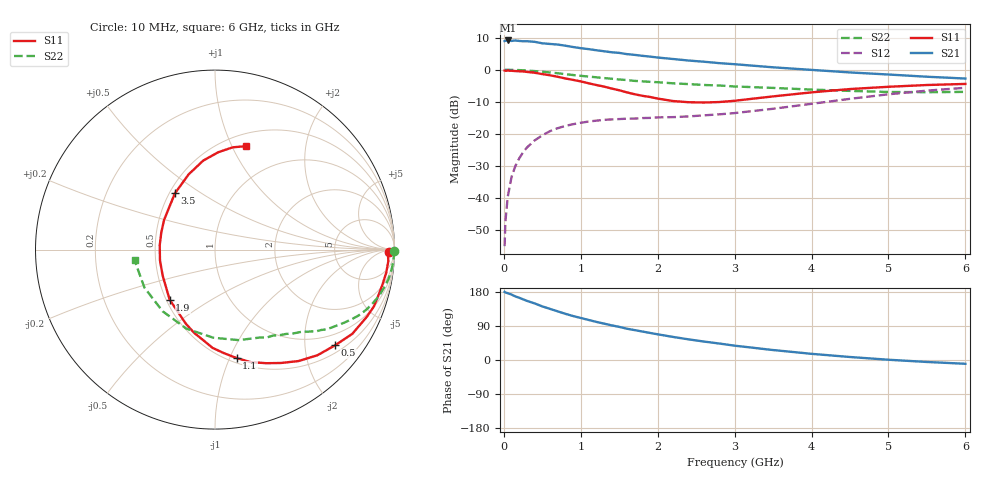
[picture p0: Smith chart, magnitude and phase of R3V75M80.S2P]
! SIEMENS Small Signal Semiconductors
! BFR181
! Si NPN RF Bipolar Junction Transistor in SOT23
! VCE = 0.75 V  IC = 0.8 mA
! Common Emitter S-Parameters:  May  1996
# GHz  S  MA  R  50
!  f  S11  S21  S12  S22
! GHz  MAG  ANG  MAG  ANG  MAG  ANG  MAG  ANG
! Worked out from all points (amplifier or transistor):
!   36 points, 10 MHz to 6 GHz, reference 50 ohm
!   highest |S21| = 9.1 dB at 50 MHz (marker M1)
!   |S21| within 3 dB of that: start of sweep to 1.189 GHz
!   unconditionally stable (mu >= 1): 2.027 GHz to 4.167 GHz
!   at 250 MHz: K = 0.15, MSG = 17.3 dB, |S12| = -25.7 dB
!   at 1.4 GHz: K = 0.74, MSG = 10.4 dB, |S12| = -15.5 dB
!   at 6 GHz: K = 0.95, MSG = 1.4 dB, |S12| = -5.6 dB
!   S11 on the Smith chart (normalised r, x): 10 MHz: 55, -25; 500 MHz: 0.68, -2.70; 1.1 GHz: 0.54, -1.06; 1.9 GHz: 0.52, -0.34; 3.5 GHz: 0.53, +0.39; 6 GHz: 0.63, +1.13
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0.01  0.9703 -0.8  2.791 179.7  0.0018 94.1  0.9983 -0.4
0.02  0.9638 -1.4  2.821 178.4  0.0043 84.0  0.9957 -0.8
0.05  0.9678 -3.8  2.852 176.2  0.0104 86.8  0.9971 -2.0
0.1  0.9627 -7.7  2.803 172.7  0.0215 84.2  0.9952 -3.9
0.15  0.9528 -12.0  2.848 167.7  0.0318 81.7  0.9907 -6.1
0.2  0.9454 -15.8  2.802 164.2  0.0418 78.9  0.9854 -7.9
0.3  0.9249 -23.9  2.776 156.1  0.0616 74.6  0.9703 -11.7
0.4  0.8977 -31.5  2.716 149.4  0.0794 69.2  0.952 -15.4
0.5  0.8554 -38.6  2.576 141.4  0.0954 64.6  0.9291 -18.7
0.7  0.7763 -53.1  2.463 128.4  0.1231 56.7  0.8809 -24.6
0.8  0.7309 -59.8  2.364 121.9  0.1337 52.9  0.8536 -27.1
1.1  0.6162 -78.7  2.092 105.8  0.1563 44.6  0.7829 -33.6
1.3  0.5473 -91.5  1.939 96.1  0.1659 40.6  0.7424 -37.1
1.6  0.444 -111.4  1.748 82.6  0.1734 36.9  0.6907 -41.5
1.9  0.3769 -132.0  1.601 71.4  0.178 35.7  0.6474 -45.8
2.2  0.3257 -153.5  1.468 60.9  0.1831 36.1  0.6144 -49.9
2.6  0.3089 175.5  1.332 48.7  0.195 38.5  0.5787 -55.8
3  0.3287 149.5  1.218 37.8  0.2116 41.1  0.5488 -63.3
3.5  0.3847 125.5  1.09 26.3  0.2469 43.3  0.5212 -75.4
4.5  0.5004 97.5  0.907 7.9  0.3524 40.6  0.4682 -110.0
5.5  0.5782 80.2  0.778 -5.2  0.4727 28.8  0.4467 -151.7
6  0.6011 73.5  0.729 -10.0  0.5238 21.2  0.4522 -172.5
